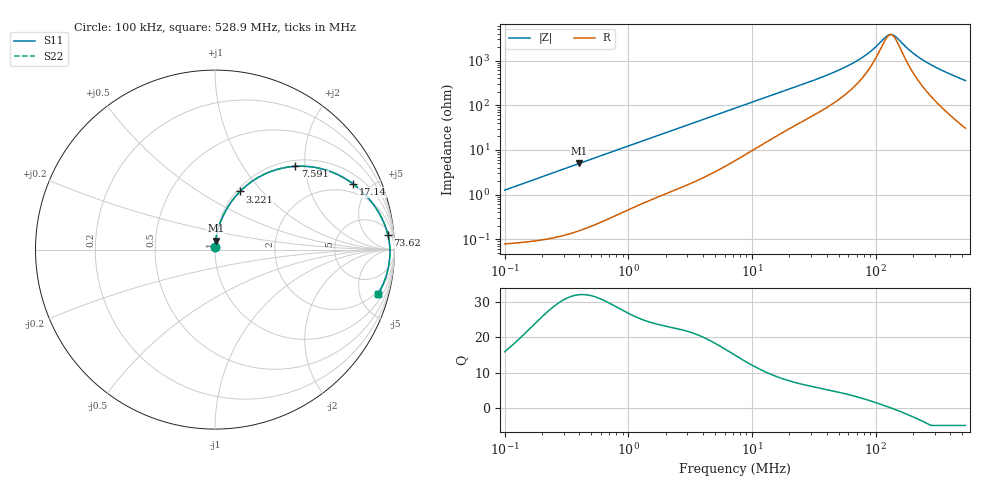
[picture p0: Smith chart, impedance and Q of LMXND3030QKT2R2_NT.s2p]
! LMXND3030QKT2R2_NT  S-PARAMETER MODEL  ( Standard Model )
! Model Generated by TAIYO YUDEN Corporation (https://www.yuden.co.jp/en/)
! Version 1.0
! TAIYO YUDEN Control No. 20250724
! Copyright(c) 2025 TAIYO YUDEN CO.,LTD. All Rights Reserved.
! Product Description (link to TY-COMPAS)
! https://ds.yuden.co.jp/TYCOMPAS/or/detail?pn=LMXND3030QKT2R2MNT&u=M
! Products Name : Inductors
! Characteristics :
!  Inductance : 2.2 [uH] , SRF(min) : 64 [MHz] , DC Resistance(max) : 0.07 [Ohm]
!  Rated Current : Saturation  1480 [m A] , Temp Rise  2200 [m A] (40 [degC])
!  Case Size : 3.0 x 3.0 / 0.118 x 0.118 [mm/inch] , Thickness : 1.5 / 0.059 [mm/inch]
!  (Conditions: Temperature = 25 [degC] , DC Bias Current = 0 [A])
! External Node Assignments :
!  1  o---GGG---o  2
! GND o---------o GND
! Frequency Range : 0.1MHz  -  528.887669MHz  [ 402 STEP ]
# MHz S RI R 50
! Freq[MHz].  S11 Real  S11 Imag  S21 Real  S21 Imag  S12 Real  S12 Imag  S22 Real  S22 Imag
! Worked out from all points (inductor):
!   401 points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, 100 kHz to 528.9 MHz, reference 50 ohm
!   read as one part in series: L = 1.98 uH near 104.4 kHz
!   highest Q = 32.1 at 402.8 kHz (marker M1), where L = 1.97 uH
!   self-resonance near 131.5 MHz
!   S11 on the Smith chart (normalised r, x): 100 kHz: 1.00, +0.02; 3.221 MHz: 1.04, +0.77; 7.591 MHz: 1.12, +1.78; 17.14 MHz: 1.47, +3.92; 73.62 MHz: 8, +20; 528.9 MHz: 1.61, -7.11
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0.1  0.000939 0.0125  0.9991 -0.0125  0.9991 -0.0125  0.000939 0.0125
0.40276  0.00402 0.0496  0.996 -0.0496  0.996 -0.0496  0.00402 0.0496
0.420401  0.0043 0.0517  0.9957 -0.0517  0.9957 -0.0517  0.0043 0.0517
0.909423  0.0161 0.1091  0.9839 -0.1091  0.9839 -0.1091  0.0161 0.1091
1.767367  0.0512 0.2003  0.9488 -0.2003  0.9488 -0.2003  0.0512 0.2003
3.220788  0.1394 0.3238  0.8606 -0.3238  0.8606 -0.3238  0.1394 0.3238
4.737111  0.2504 0.4075  0.7496 -0.4075  0.7496 -0.4075  0.2504 0.4075
7.430023  0.4371 0.4633  0.5629 -0.4633  0.5629 -0.4633  0.4371 0.4633
7.590992  0.4468 0.464  0.5532 -0.464  0.5532 -0.464  0.4468 0.464
10.92802  0.6099 0.4458  0.3901 -0.4458  0.3901 -0.4458  0.6099 0.4458
17.14029  0.7704 0.3654  0.2296 -0.3654  0.2296 -0.3654  0.7704 0.3654
30.5735  0.8911 0.2397  0.1089 -0.2397  0.1089 -0.2397  0.8911 0.2397
51.13837  0.9442 0.1423  0.0558 -0.1423  0.0558 -0.1423  0.9442 0.1423
73.61899  0.9633 0.0832  0.0367 -0.0832  0.0367 -0.0832  0.9633 0.0832
89.28233  0.9692 0.0546  0.0308 -0.0546  0.0308 -0.0546  0.9692 0.0546
117.9709  0.9739 0.0151  0.0261 -0.0151  0.0261 -0.0151  0.9739 0.0151
128.5312  0.9745 0.00315  0.0255 -0.00315  0.0255 -0.00315  0.9745 0.00315
143.0706  0.9748 -0.0119  0.0252 0.0119  0.0252 0.0119  0.9748 -0.0119
193.1382  0.9726 -0.0552  0.0274 0.0552  0.0274 0.0552  0.9726 -0.0552
255.1982  0.9659 -0.0994  0.0341 0.0994  0.0341 0.0994  0.9659 -0.0994
359.5937  0.9486 -0.1624  0.0514 0.1624  0.0514 0.1624  0.9486 -0.1624
528.8877  0.9089 -0.248  0.0911 0.248  0.0911 0.248  0.9089 -0.248
